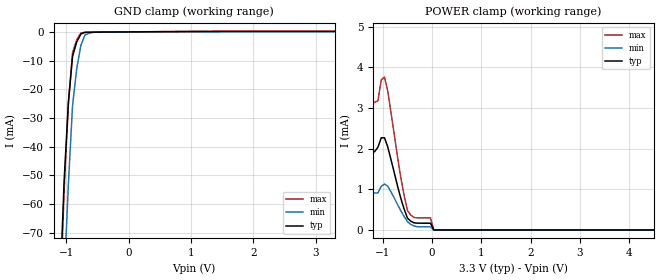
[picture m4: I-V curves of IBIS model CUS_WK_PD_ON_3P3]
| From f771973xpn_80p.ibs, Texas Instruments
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|   Model Cell CUS_WK_PD_ON_3P3
|CUS_WK_PD_ON_3P3
[Model]   CUS_WK_PD_ON_3P3
Model_type   Input
Polarity   Non-Inverting
Vinl =  0.8
Vinh =  2
C_comp   2.12034p   1.0392p   2.53442p
[Model Spec]
Vinl   0.8   0.8   0.8
Vinh   2   2   2
[Temperature Range]   25   155   -40
[Voltage Range]   3.3   2.97   3.63
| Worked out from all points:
|   GND clamp passes 1 mA (typ) near -0.77 V on its own axis
|   POWER clamp passes 1 mA (typ) near -0.68 V on its own axis
| Nom Voltages:
|   BIASFET=3.3, VDD=1.2, VDDS=3.3, VSS=0
| Min Voltages:
|   BIASFET=2.97, VDD=1.08, VDDS=2.97, VSS=0
| Max Voltages:
|   BIASFET=3.63, VDD=1.32, VDDS=3.63, VSS=0
[POWER_clamp]
|   voltage   I(typ)   I(min)   I(max)
-3.3V     2.313mA    637.4mA    3.948mA
-2.167V   1.926mA    7.214mA    3.281mA
-2.1V     1.919mA    1.782mA    3.261mA
-1.967V   1.908mA    961.4uA    3.226mA
-1.167V   1.929mA    911.7uA    3.138mA
-966.7mV  2.267mA    1.129mA    3.762mA
-566.7mV  508.5uA    327.8uA    838uA
-500mV    290.5uA    203.5uA    476.4uA
-366.7mV  175.3uA    96.24uA    306.9uA
-33.33mV  167uA      77.21uA    297.4uA
33.33mV   0A         0A         0A
6.6V      0A         0A         0A
[GND_clamp]
|   voltage   I(typ)   I(min)   I(max)
-3.3V     -2.204A    -1.834A    -3.186A
-1.1V     -88.85mA   -124.4mA   -95.55mA
-1.033V   -51.38mA   -86.06mA   -54.51mA
-966.7mV  -24.61mA   -53.17mA   -25.09mA
-900mV    -8.554mA   -25.73mA   -7.279mA
-833.3mV  -3.532mA   -12.91mA   -2.741mA
-766.7mV  -729.8uA   -4.685mA   -370.7uA
-700mV    -146.6uA   -1.063mA   -167.8uA
-566.7mV  -87.36uA   -126.3uA   -131.5uA
3.3V      167uA      83.52uA    297.2uA
